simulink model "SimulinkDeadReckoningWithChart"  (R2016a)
settings: Solver=FixedStepAuto  StartTime=0.0  StopTime=inf  RelTol=1e-3
libraries: miniQ x1

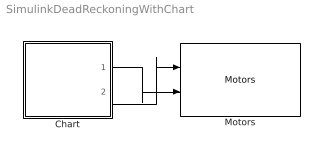
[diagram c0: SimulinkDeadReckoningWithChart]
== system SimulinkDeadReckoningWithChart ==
  Chart : Stateflow chart  TreatAsAtomicUnit=on
  Motors : miniQ/Motors  flipLeft=off  flipRight=off
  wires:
  Chart/2(l) -> Motors/1
  Chart/1(r) -> Motors/2

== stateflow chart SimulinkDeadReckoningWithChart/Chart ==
  state Experiment with changing the "after(int,sec) function and also the values for r and l to get the dead reckoing patter you desire [group]
  state Forward
    entry: r=255
    l=255
  state Right
    entry: r=-255
    l=255
  state Forward2
    entry: r=255
    l=255
  state Stop
    entry: r=0
    l=0
  state Left
    entry: r=255
    l=-255
  state Forward1
    entry: r=255
    l=255
  (default) -> Forward
  Forward2 -> Stop : after(2,sec)
  Right -> Forward2 : after(1,sec)
  Forward -> Left : after(2,sec)
  Forward1 -> Right : after(1,sec)
  Left -> Forward1 : after(1,sec)
  data: r output; l output
